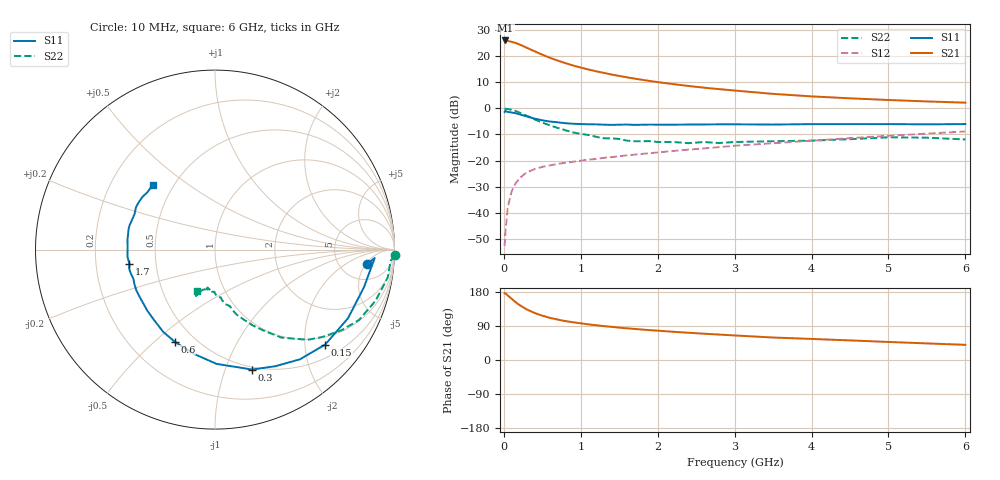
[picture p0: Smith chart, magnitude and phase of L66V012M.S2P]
!  INFINEON TECHNOLOGIES Small Signal Semiconductors
! BFR380L3 , Si-NPN RF-Transistor in TSLP-3-1
!  Vce=6 V,  Ic=12.5 mA
! Common Emitter S-Parameters:  07. March 2005
#  GHz  S  MA  R  50
! f  S11  S21  S12  S22
! GHz  Mag  Ang  Mag  Ang  Mag  Ang  Mag  Ang
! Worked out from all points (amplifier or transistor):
!   36 points, 10 MHz to 6 GHz, reference 50 ohm
!   highest |S21| = 26.0 dB at 20 MHz (marker M1)
!   |S21| within 3 dB of that: start of sweep to 312.7 MHz
!   unconditionally stable (mu >= 1): 2.667 GHz to 4.623 GHz
!   at 250 MHz: K = 0.23, MSG = 24.7 dB, |S12| = -25.6 dB
!   at 1.4 GHz: K = 0.83, MSG = 15.8 dB, |S12| = -18.7 dB
!   at 6 GHz: K = 0.96, MSG = 5.5 dB, |S12| = -8.8 dB
!   S11 on the Smith chart (normalised r, x): 10 MHz: 9, -5; 150 MHz: 0.80, -2.46; 300 MHz: 0.47, -1.24; 600 MHz: 0.39, -0.58; 1.7 GHz: 0.35, -0.07; 6 GHz: 0.39, +0.37
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0.01  0.853 -5.3  19.89 176.1  0.0023 74.0  1.003 -1.8
0.02  0.8911 -3.0  19.97 176.2  0.0041 82.7  0.9803 -3.7
0.05  0.8562 -14.1  19.59 170.5  0.0126 83.0  0.9749 -9.1
0.1  0.8341 -27.3  18.82 161.7  0.0254 75.8  0.9389 -17.7
0.15  0.8103 -40.8  17.96 153.2  0.0362 70.3  0.8933 -26.0
0.2  0.7729 -52.3  16.8 145.6  0.0452 65.7  0.8371 -32.4
0.25  0.7317 -62.6  15.61 139.3  0.0527 60.7  0.7736 -38.9
0.3  0.6995 -72.8  14.41 133.3  0.0596 57.7  0.7209 -44.2
0.4  0.6368 -89.2  12.37 124.0  0.0688 52.9  0.6148 -52.9
0.5  0.5911 -102.2  10.68 117.0  0.0758 50.4  0.5343 -58.4
0.6  0.56 -113.7  9.289 111.1  0.0811 48.5  0.4726 -63.5
0.7  0.5413 -122.3  8.219 106.7  0.0863 48.1  0.4221 -67.6
0.8  0.5198 -130.4  7.352 102.7  0.091 47.7  0.3817 -71.6
1.1  0.4957 -147.9  5.549 94.0  0.1043 49.5  0.3094 -79.1
1.4  0.4826 -160.3  4.448 87.5  0.1164 51.1  0.2665 -84.5
1.7  0.4832 -170.4  3.712 82.0  0.1301 52.8  0.2347 -90.8
2.2  0.4872 178.1  2.915 74.5  0.1528 55.4  0.2273 -96.4
2.8  0.4948 166.6  2.333 67.1  0.1812 57.8  0.217 -104.0
3.5  0.49 156.3  1.895 59.3  0.215 58.2  0.2348 -107.3
4.5  0.5003 148.6  1.557 51.7  0.2691 59.3  0.2572 -110.3
5.5  0.494 139.5  1.358 43.8  0.3285 57.8  0.275 -112.6
6  0.5008 133.8  1.286 40.0  0.361 56.4  0.2537 -113.3
